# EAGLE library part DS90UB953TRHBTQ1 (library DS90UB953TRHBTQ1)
2 MP MIPI CSI-2 FPD-Link III serializer for 2MP/60fps cameras & radar Source: Datasheet
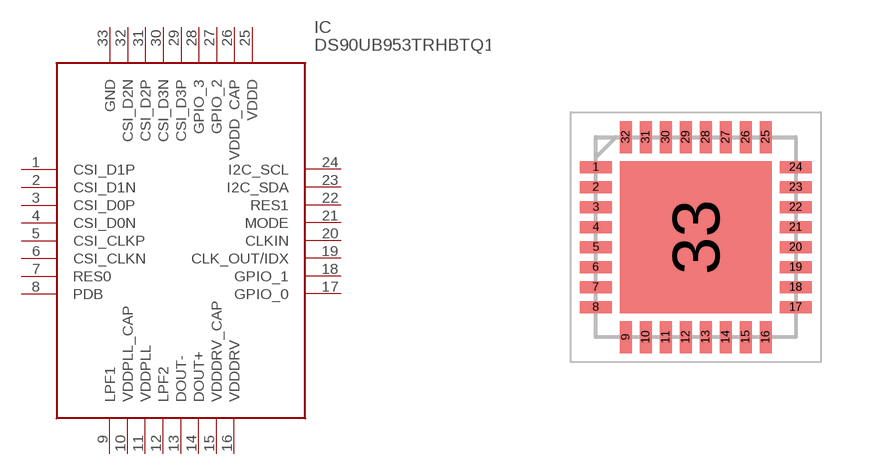
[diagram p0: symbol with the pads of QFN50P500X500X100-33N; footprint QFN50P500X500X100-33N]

Designator prefix IC

## DS90UB953TRHBTQ1 (Description: 2 MP MIPI CSI-2 FPD-Link III serializer for 2MP/60fps cameras & radar; Height: 1mm; Manufacturer_Name: Texas Instruments; Manufacturer_Part_Number: DS90UB953TRHBTQ1; Mouser_Part_Number: 595-DS90UB953TRHBTQ1; Mouser_Price-Stock: https://www.mouser.co.uk/ProductDetail/Texas-Instruments/DS90UB953TRHBTQ1?qs=OEYMhS7p3YYobKAcq0j91Q%3D%3D)  [QFN50P500X500X100-33N]
1  CSI_D1P
2  CSI_D1N
3  CSI_D0P
4  CSI_D0N
5  CSI_CLKP
6  CSI_CLKN
7  RES0
8  PDB
9  LPF1
10  VDDPLL_CAP
11  VDDPLL
12  LPF2
13  DOUT-
14  DOUT+
15  VDDDRV_CAP
16  VDDDRV
17  GPIO_0
18  GPIO_1
19  CLK_OUT/IDX
20  CLKIN
21  MODE
22  RES1
23  I2C_SDA
24  I2C_SCL
25  VDDD
26  VDDD_CAP
27  GPIO_2
28  GPIO_3
29  CSI_D3P
30  CSI_D3N
31  CSI_D2P
32  CSI_D2N
33  GND

## Footprint QFN50P500X500X100-33N (pad centres in mm)
RHB0032P vqfn
smd 0.8 x 0.3: 1 -2.5,1.75; 2 -2.5,1.25; 3 -2.5,0.75; 4 -2.5,0.25; 5 -2.5,-0.25; 6 -2.5,-0.75; 7 -2.5,-1.25; 8 -2.5,-1.75; 17 2.5,-1.75; 18 2.5,-1.25; 19 2.5,-0.75; 20 2.5,-0.25; 21 2.5,0.25; 22 2.5,0.75; 23 2.5,1.25; 24 2.5,1.75
smd 0.3 x 0.8: 9 -1.75,-2.5; 10 -1.25,-2.5; 11 -0.75,-2.5; 12 -0.25,-2.5; 13 0.25,-2.5; 14 0.75,-2.5; 15 1.25,-2.5; 16 1.75,-2.5; 25 1.75,2.5; 26 1.25,2.5; 27 0.75,2.5; 28 0.25,2.5; 29 -0.25,2.5; 30 -0.75,2.5; 31 -1.25,2.5; 32 -1.75,2.5
smd 3.8 x 3.8: 33 0,0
